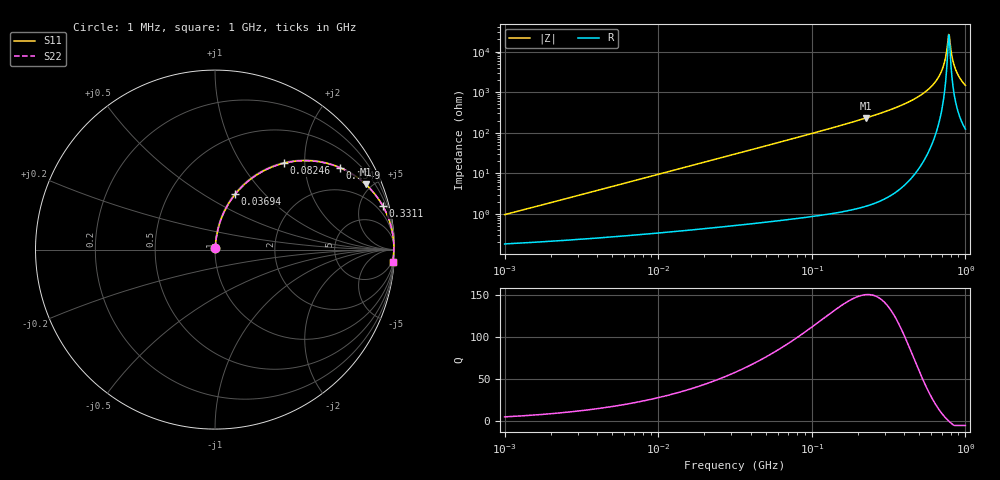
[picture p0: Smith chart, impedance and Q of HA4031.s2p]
# MHz S MA R 50
!Freq  MagS11  AngS11  MagS21  AngS21  MagS12  AngS12  MagS22  AngS22
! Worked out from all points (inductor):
!   801 points, 1 MHz to 1 GHz, reference 50 ohm
!   read as one part in series: L = 150 nH near 1.035 MHz
!   highest Q = 150 at 224.5 MHz (marker M1), where L = 164 nH
!   self-resonance near 778.5 MHz
!   S11 on the Smith chart (normalised r, x): 1 MHz: 1.00, +0.02; 36.94 MHz: 1.01, +0.70; 82.46 MHz: 1.02, +1.57; 154.9 MHz: 1.02, +3.04; 331.1 MHz: 1.06, +7.61; 1 GHz: 3, -29
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1  0.009581 78.5  0.9981 -0.5  0.9981 -0.5  0.009581 78.5
3.180534  0.02999 83.7  0.9972 -1.7  0.9972 -1.7  0.02999 83.7
10.02882  0.09386 82.6  0.9922 -5.4  0.9922 -5.4  0.09386 82.6
31.89701  0.287 72.3  0.953 -16.7  0.953 -16.7  0.287 72.3
36.94026  0.3279 70.0  0.9396 -19.1  0.9396 -19.1  0.3279 70.0
82.46127  0.615 51.5  0.7824 -37.9  0.7824 -37.9  0.615 51.5
100.5773  0.6909 45.8  0.7168 -43.7  0.7168 -43.7  0.6909 45.8
154.8817  0.8326 33.2  0.5479 -56.4  0.5479 -56.4  0.8326 33.2
224.5174  0.9153 23.4  0.3968 -66.2  0.3968 -66.2  0.9153 23.4
317.1393  0.9613 15.6  0.2686 -74.0  0.2686 -74.0  0.9613 15.6
331.1311  0.9653 14.7  0.2537 -74.9  0.2537 -74.9  0.9653 14.7
484.1724  0.989 7.7  0.1334 -81.5  0.1334 -81.5  0.989 7.7
616.595  0.9953 3.7  0.06455 -84.0  0.06455 -84.0  0.9953 3.7
701.8592  0.9965 1.7  0.02914 -82.2  0.02914 -82.2  0.9965 1.7
732.8245  0.9965 1.0  0.01757 -78.1  0.01757 -78.1  0.9965 1.0
765.156  0.9964 0.3  0.006597 -57.0  0.006597 -57.0  0.9964 0.3
778.4846  0.9963 0.1  0.003766 -13.5  0.003766 -13.5  0.9963 0.1
798.9139  0.9962 -0.4  0.007222 57.7  0.007222 57.7  0.9962 -0.4
834.1612  0.9957 -1.0  0.01828 76.0  0.01828 76.0  0.9957 -1.0
870.9636  0.9951 -1.7  0.02984 79.8  0.02984 79.8  0.9951 -1.7
933.2543  0.9938 -2.8  0.04856 81.3  0.04856 81.3  0.9938 -2.8
1000  0.9921 -3.9  0.06747 81.3  0.06747 81.3  0.9921 -3.9
